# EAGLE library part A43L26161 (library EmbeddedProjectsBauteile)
1M x 16Bit x 4 Banks SDRAM
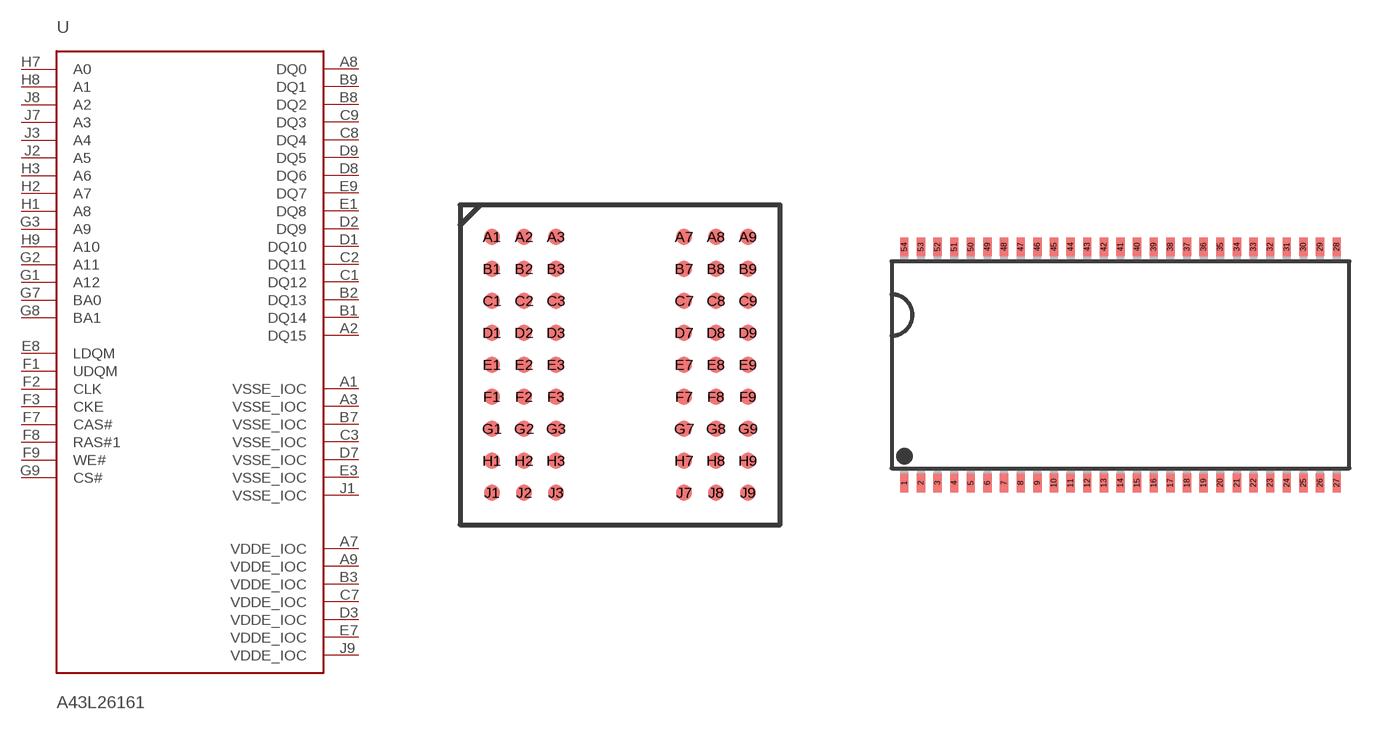
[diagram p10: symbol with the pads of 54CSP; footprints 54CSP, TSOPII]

Designator prefix -

## A43L26161  [54CSP]
A1  VSSE_IOC  pwr
A2  DQ15
A3  VSSE_IOC  pwr
A7  VDDE_IOC  pwr
A8  DQ0
A9  VDDE_IOC  pwr
B1  DQ14
B2  DQ13
B3  VDDE_IOC  pwr
B7  VSSE_IOC  pwr
B8  DQ2
B9  DQ1
C1  DQ12
C2  DQ11
C3  VSSE_IOC  pwr
C7  VDDE_IOC  pwr
C8  DQ4
C9  DQ3
D1  DQ10
D2  DQ9
D3  VDDE_IOC  pwr
D7  VSSE_IOC  pwr
D8  DQ6
D9  DQ5
E1  DQ8
E3  VSSE_IOC  pwr
E7  VDDE_IOC  pwr
E8  LDQM
E9  DQ7
F1  UDQM
F2  CLK
F3  CKE
F7  CAS#
F8  RAS#1
F9  WE#
G1  A12
G2  A11
G3  A9
G7  BA0
G8  BA1
G9  CS#
H1  A8
H2  A7
H3  A6
H7  A0
H8  A1
H9  A10
J1  VSSE_IOC  pwr
J2  A5
J3  A4
J7  A3
J8  A2
J9  VDDE_IOC  pwr

## A43L26161TSOPII (EP: 400486)  [TSOPII]
1  VDDE_IOC  pwr
2  DQ0
3  VDDE_IOC  pwr
4  DQ1
5  DQ2
6  VSSE_IOC  pwr
7  DQ3
8  DQ4
9  VDDE_IOC  pwr
10  DQ5
11  DQ6
12  VSSE_IOC  pwr
13  DQ7
14  VDDE_IOC  pwr
15  LDQM
16  WE#
17  CAS#
18  RAS#1
19  CS#
20  BA0
21  BA1
22  A10
23  A0
24  A1
25  A2
26  A3
27  VDDE_IOC  pwr
28  VSSE_IOC  pwr
29  A4
30  A5
31  A6
32  A7
33  A8
34  A9
35  A11
36  A12
37  CKE
38  CLK
39  UDQM
41  VSSE_IOC  pwr
42  DQ8
43  VDDE_IOC  pwr
44  DQ9
45  DQ10
46  VSSE_IOC  pwr
47  DQ11
48  DQ12
49  VDDE_IOC  pwr
50  DQ13
51  DQ14
52  VSSE_IOC  pwr
53  DQ15
54  VSSE_IOC  pwr

## Footprint 54CSP (pad centres in mm)
smd 0.4 x 0.4: A1 -3.2,3.2; A2 -2.4,3.2; A3 -1.6,3.2; A7 1.6,3.2; A8 2.4,3.2; A9 3.2,3.2; B1 -3.2,2.4; B2 -2.4,2.4; B3 -1.6,2.4; B7 1.6,2.4; B8 2.4,2.4; B9 3.2,2.4; C1 -3.2,1.6; C2 -2.4,1.6; C3 -1.6,1.6; C7 1.6,1.6; C8 2.4,1.6; C9 3.2,1.6; D1 -3.2,0.8; D2 -2.4,0.8; D3 -1.6,0.8; D7 1.6,0.8; D8 2.4,0.8; D9 3.2,0.8; E1 -3.2,0; E2 -2.4,0; E3 -1.6,0; E7 1.6,0; E8 2.4,0; E9 3.2,0; F1 -3.2,-0.8; F2 -2.4,-0.8; F3 -1.6,-0.8; F7 1.6,-0.8; F8 2.4,-0.8; F9 3.2,-0.8; G1 -3.2,-1.6; G2 -2.4,-1.6; G3 -1.6,-1.6; G7 1.6,-1.6; G8 2.4,-1.6; G9 3.2,-1.6; H1 -3.2,-2.4; H2 -2.4,-2.4; H3 -1.6,-2.4; H7 1.6,-2.4; H8 2.4,-2.4; H9 3.2,-2.4; J1 -3.2,-3.2; J2 -2.4,-3.2; J3 -1.6,-3.2; J7 1.6,-3.2; J8 2.4,-3.2; J9 3.2,-3.2

## Footprint TSOPII (pad centres in mm)
smd 0.4 x 0.9: 1 -10.4,-5.68; 2 -9.6,-5.68; 3 -8.8,-5.68; 4 -8,-5.68; 5 -7.2,-5.68; 6 -6.4,-5.68; 7 -5.6,-5.68; 8 -4.8,-5.68; 9 -4,-5.68; 10 -3.2,-5.68; 11 -2.4,-5.68; 12 -1.6,-5.68; 13 -0.8,-5.68; 14 0,-5.68; 15 0.8,-5.68; 16 1.6,-5.68; 17 2.4,-5.68; 18 3.2,-5.68; 19 4,-5.68; 20 4.8,-5.68; 21 5.6,-5.68; 22 6.4,-5.68; 23 7.2,-5.68; 24 8,-5.68; 25 8.8,-5.68; 26 9.6,-5.68; 27 10.4,-5.68; 28 10.4,5.68; 29 9.6,5.68; 30 8.8,5.68; 31 8,5.68; 32 7.2,5.68; 33 6.4,5.68; 34 5.6,5.68; 35 4.8,5.68; 36 4,5.68; 37 3.2,5.68; 38 2.4,5.68; 39 1.6,5.68; 40 0.8,5.68; 41 0,5.68; 42 -0.8,5.68; 43 -1.6,5.68; 44 -2.4,5.68; 45 -3.2,5.68; 46 -4,5.68; 47 -4.8,5.68; 48 -5.6,5.68; 49 -6.4,5.68; 50 -7.2,5.68; 51 -8,5.68; 52 -8.8,5.68; 53 -9.6,5.68; 54 -10.4,5.68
